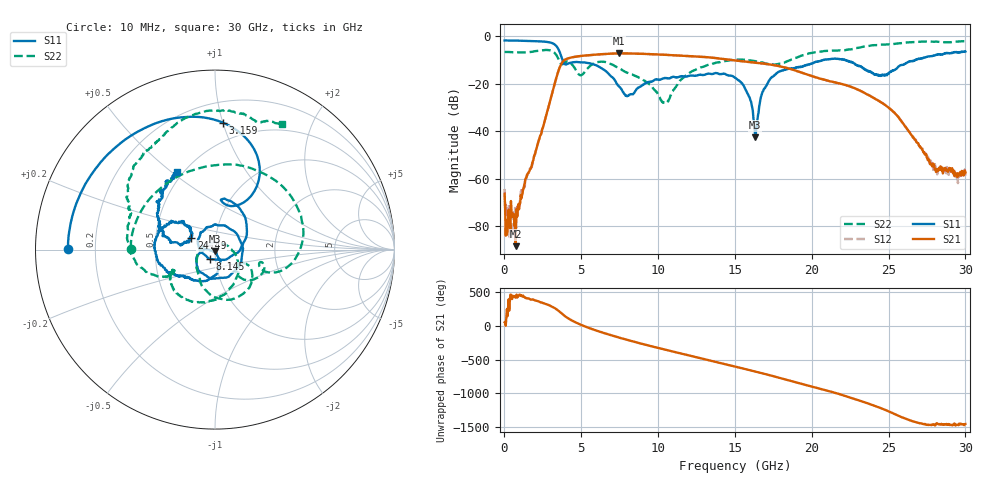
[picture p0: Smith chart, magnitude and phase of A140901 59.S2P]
!  2-Port S-parameters saved by WinCal
! VAR MeasName=S-Parameters (CALIBRATED_DATA) read from VNA (N5244A)
! VAR MeasDate=11/3/2014 9:36:32 AM
! VAR NAME=A140901 59
! VAR FILENAME=A140901 59.S2P
! VAR DATE=11/3/2014 9:36:32 AM
! VAR PHYS_PORTS=1,2
# Hz S RI R 50
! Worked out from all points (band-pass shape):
!   801 points, 10 MHz to 30 GHz, reference 50 ohm
!   highest |S21| = -7.16 dB at 7.433 GHz (marker M1); lowest = -88.3 dB at 722.3 MHz (marker M2)
!   |S21| within 3 dB of the highest: 3.87 GHz to 15.04 GHz (11.17 GHz wide, 118 % of centre)
!   lowest |S11| = -42.6 dB at 16.32 GHz (marker M3), VSWR 1.01, Z = 49.9 - j0.729 ohm
!   |S11| at or under -10 dB: 3.782 GHz to 20.73 GHz (16.95 GHz wide, 138 % of centre); 22.2 GHz to 26.73 GHz (4.526 GHz wide, 18.5 % of centre)
!   |S22| runs from -28.0 to -2.0 dB; largest |S21 - S12| = 0.0035
!   S11 on the Smith chart (normalised r, x): 10 MHz: 0.10, +0.00; 3.159 GHz: 0.35, +1.00; 8.145 GHz: 0.94, -0.10; 24.49 GHz: 0.76, +0.10; 30 GHz: 0.47, +0.52
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1e7  -0.8192 0.00339  0.000268 0.000402  -0.00017 0.00059  -0.4689 0.00533
3.84875e8  -0.8082 0.1252  -1.72e-05 6.42e-05  -2.56e-05 0.000104  -0.4324 0.1734
7.222625e8  -0.7813 0.2324  1.85e-05 3.36e-05  8.42e-05 0.000153  -0.3514 0.2968
2.1093e9  -0.4911 0.6195  0.00453 0.00109  0.00454 0.00108  0.171 0.4615
3.15895e9  0.0436 0.7076  0.0138 -0.0724  0.0139 -0.0725  0.4782 0.0122
3.871212e9  0.1206 0.2465  -0.2882 0.1158  -0.2876 0.1155  0.2627 -0.071
5.033325e9  0.0794 0.2723  0.3797 0.0851  0.3793 0.0851  0.1313 -0.0813
6.232925e9  0.1759 0.1342  0.0249 -0.4192  0.0253 -0.4185  0.1415 -0.2558
7.432525e9  0.0775 -0.0468  -0.4323 -0.0723  -0.4316 -0.0726  -0.0718 -0.2031
8.144788e9  -0.0269 -0.0528  -0.3534 0.257  -0.353 0.2564  -0.0927 -0.1346
1.001916e10  -0.0714 0.0999  0.3479 0.2272  0.3471 0.2269  -0.0553 0.0224
1.223092e10  0.1259 0.0808  0.00264 -0.3802  0.00237 -0.38  0.1294 -0.1341
1.361796e10  0.0914 -0.1363  -0.3434 -0.0816  -0.3433 -0.0821  0.0188 -0.2675
1.5005e10  -0.1004 -0.0889  -0.1414 0.2774  -0.1399 0.2769  -0.1575 -0.2796
1.59047e10  -0.0546 0.0027  0.1106 0.2666  0.1095 0.2666  -0.2392 -0.2046
1.631706e10  -0.00137 -0.00731  0.2015 0.1925  0.1987 0.1946  -0.2503 -0.1678
1.736671e10  0.00979 -0.1337  0.2414 -0.0772  0.242 -0.0761  -0.2301 -0.1156
2.002832e10  -0.234 -0.1337  -0.1451 0.00515  -0.1457 0.0043  -0.444 -0.0643
2.448934e10  -0.1311 0.0658  -0.0317 -0.0264  -0.0315 -0.0268  -0.3917 0.5395
2.501416e10  -0.1582 0.0406  -0.0308 0.00515  -0.0311 0.00505  -0.331 0.5955
2.808814e10  -0.317 0.2599  0.00137 -0.000259  0.0015 -0.000592  0.1586 0.7585
3e10  -0.2096 0.4297  0.00131 -0.000371  0.00112 -0.000361  0.3756 0.7004
